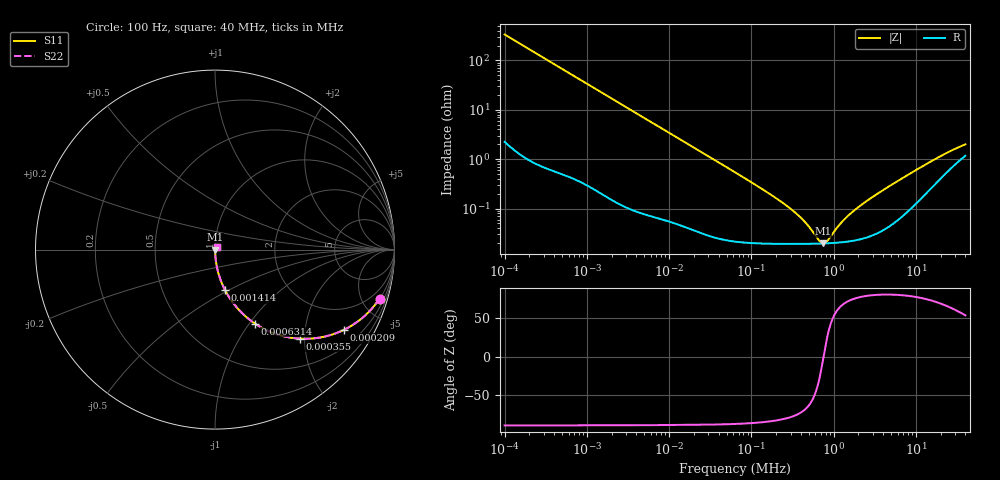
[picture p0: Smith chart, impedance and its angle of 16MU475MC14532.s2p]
!Components F PML CAP
!CONCATENATE F 0.1-40000kHz, at 20deg DC=0V
!Part Number F 16MU475MC14532
!Copyright(C) Rubycon Corporation. 20161128
# MHz S MA R 50
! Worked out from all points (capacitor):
!   561 points, 100 Hz to 40 MHz, reference 50 ohm
!   read as one part in series: C = 4.75 uF near 104.7 Hz
!   lowest |Z| = 19.7 mohm at 743.7 kHz (marker M1)
!   series resonance near 753.9 kHz, so ESL is about 9.4 nH
!   S11 on the Smith chart (normalised r, x): 100 Hz: 1.04, -6.70; 209 Hz: 1.02, -3.21; 355 Hz: 1.01, -1.89; 631.4 Hz: 1.01, -1.07; 1.414 kHz: 1.00, -0.48; 40 MHz: 1.02, +0.03
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0.0001  0.9565 -16.6  0.2853 73.0  0.2853 73.0  0.9565 -16.6
0.0001445636  0.9163 -23.3  0.3951 66.4  0.3951 66.4  0.9163 -23.3
0.0002089863  0.8466 -31.8  0.5275 57.8  0.5275 57.8  0.8466 -31.8
0.0003549787  0.685 -46.4  0.7242 43.2  0.7242 43.2  0.685 -46.4
0.000631385  0.4689 -61.6  0.8795 28.0  0.8795 28.0  0.4689 -61.6
0.0008716573  0.3598 -68.4  0.9299 21.1  0.9299 21.1  0.3598 -68.4
0.001413914  0.2322 -76.1  0.9706 13.4  0.9706 13.4  0.2322 -76.1
0.00302374  0.1114 -83.1  0.9927 6.4  0.9927 6.4  0.1114 -83.1
0.007424854  0.04582 -86.6  0.9983 2.6  0.9983 2.6  0.04582 -86.6
0.06324555  0.005432 -87.4  0.9998 0.3  0.9998 0.3  0.005432 -87.4
0.2699366  0.001134 -80.2  0.9998 0.1  0.9998 0.1  0.001134 -80.2
0.4086278  0.0006264 -72.1  0.9998 0.0  0.9998 0.0  0.0006264 -72.1
0.5512845  0.0003495 -56.3  0.9998 0.0  0.9998 0.0  0.0003495 -56.3
0.6628347  0.0002298 -31.9  0.9998 0.0  0.9998 0.0  0.0002298 -31.9
0.7437442  0.0001966 -3.8  0.9998 0.0  0.9998 0.0  0.0001966 -3.8
0.8345301  0.0002182 25.0  0.9998 -0.0  0.9998 -0.0  0.0002182 25.0
1.178955  0.0004706 64.1  0.9998 -0.0  0.9998 -0.0  0.0004706 64.1
1.66553  0.0008325 74.6  0.9998 -0.0  0.9998 -0.0  0.0008325 74.6
2.521265  0.001425 79.5  0.9997 -0.1  0.9997 -0.1  0.001425 79.5
4.69589  0.0028 81.1  0.9996 -0.2  0.9996 -0.2  0.0028 81.1
16.28983  0.009588 72.3  0.9971 -0.5  0.9971 -0.5  0.009588 72.3
40  0.01987 53.5  0.9883 -0.9  0.9883 -0.9  0.01987 53.5
